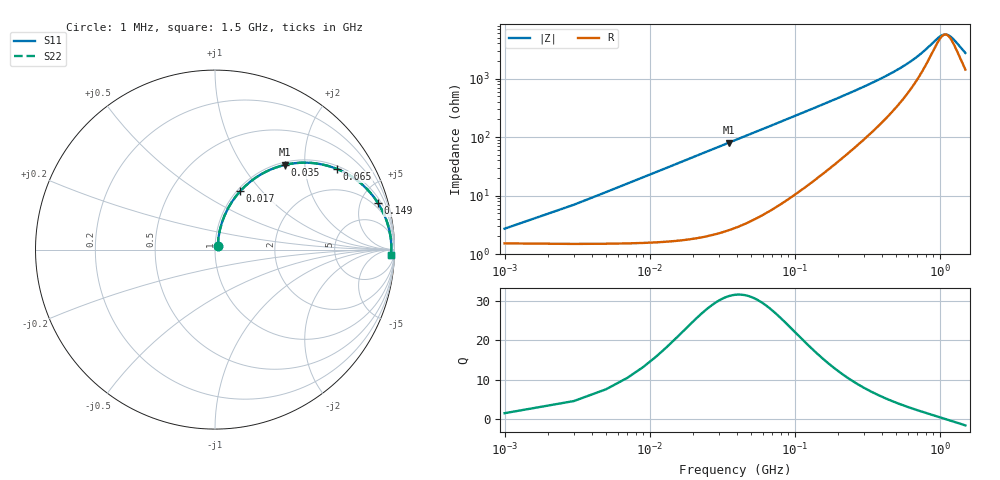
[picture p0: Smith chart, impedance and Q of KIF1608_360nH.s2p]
# MHz S RI R 50
!Freq ReS11 ImS11 ReS21 ImS21 ReS12 ImS12 ReS22 ImS22
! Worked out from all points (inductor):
!   751 points, 1 MHz to 1.5 GHz, reference 50 ohm
!   read as one part in series: L = 362 nH near 7 MHz
!   highest Q = 31.2 at 35 MHz (marker M1), where L = 362 nH
!   self-resonance near 1.094 GHz
!   S11 on the Smith chart (normalised r, x): 1 MHz: 1.03, +0.04; 17 MHz: 1.03, +0.77; 35 MHz: 1.05, +1.59; 65 MHz: 1.10, +2.96; 149 MHz: 1.43, +6.87; 1.5 GHz: 29, -47
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1  0.0155 0.0218  0.9845 -0.0218  0.9845 -0.0218  0.0155 0.0218
5  0.027 0.1089  0.973 -0.1089  0.973 -0.1089  0.027 0.1089
9  0.0537 0.1906  0.9463 -0.1906  0.9463 -0.1906  0.0537 0.1906
13  0.0927 0.2639  0.9073 -0.2639  0.9073 -0.2639  0.0927 0.2639
17  0.141 0.3264  0.859 -0.3264  0.859 -0.3264  0.141 0.3264
25  0.2521 0.4168  0.7479 -0.4168  0.7479 -0.4168  0.2521 0.4168
35  0.3917 0.4724  0.6083 -0.4724  0.6083 -0.4724  0.3917 0.4724
49  0.5531 0.4814  0.4469 -0.4814  0.4469 -0.4814  0.5531 0.4814
65  0.6815 0.4487  0.3185 -0.4487  0.3185 -0.4487  0.6815 0.4487
81  0.7653 0.4047  0.2347 -0.4047  0.2347 -0.4047  0.7653 0.4047
99  0.8263 0.3571  0.1737 -0.3571  0.1737 -0.3571  0.8263 0.3571
149  0.9085 0.2588  0.0915 -0.2588  0.0915 -0.2588  0.9085 0.2588
251  0.9573 0.1568  0.0427 -0.1568  0.0427 -0.1568  0.9573 0.1568
357  0.9716 0.106  0.0284 -0.106  0.0284 -0.106  0.9716 0.106
501  0.9785 0.0679  0.0215 -0.0679  0.0215 -0.0679  0.9785 0.0679
751  0.9821 0.0311  0.0179 -0.0311  0.0179 -0.0311  0.9821 0.0311
917  0.9827 0.0146  0.0173 -0.0146  0.0173 -0.0146  0.9827 0.0146
1001  0.9827 0.00745  0.0173 -0.00745  0.0173 -0.00745  0.9827 0.00745
1059  0.9827 0.00276  0.0173 -0.00276  0.0173 -0.00276  0.9827 0.00276
1115  0.9826 -0.00161  0.0174 0.00161  0.0174 0.00161  0.9826 -0.00161
1251  0.9821 -0.0118  0.0179 0.0118  0.0179 0.0118  0.9821 -0.0118
1500  0.9804 -0.0301  0.0196 0.0301  0.0196 0.0301  0.9804 -0.0301
